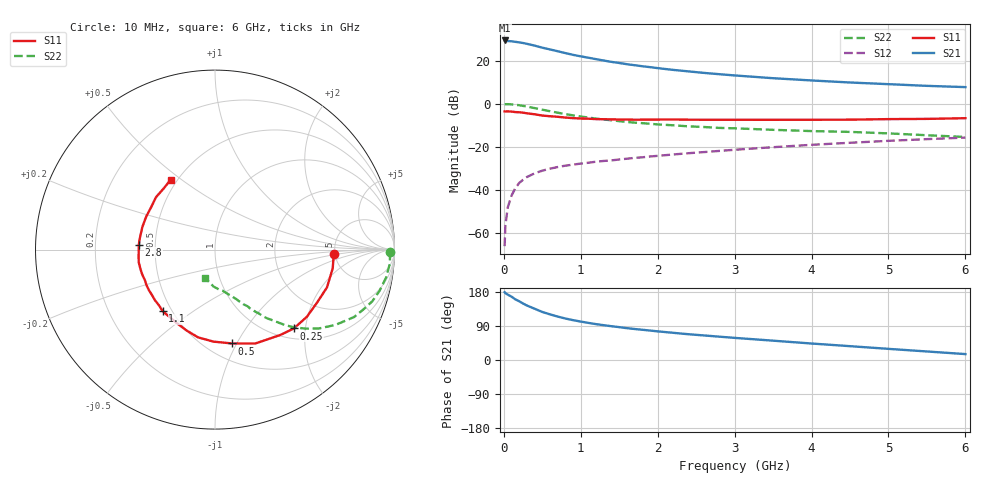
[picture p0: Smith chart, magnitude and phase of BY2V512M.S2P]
! SIEMENS Small Signal Semiconductors
! BFY420
! Si NPN RF SIEGET Grounded Emitter Transistor in MICRO-X
! VCE = 2.5 V  IC = 12 mA
! Common Emitter S-Parameters:  October  1996
# GHz  S  MA  R  50
!  f  S11  S21  S12  S22
! GHz  MAG  ANG  MAG  ANG  MAG  ANG  MAG  ANG
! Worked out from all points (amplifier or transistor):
!   36 points, 10 MHz to 6 GHz, reference 50 ohm
!   highest |S21| = 29.3 dB at 10 MHz (marker M1)
!   |S21| within 3 dB of that: start of sweep to 463.6 MHz
!   unconditionally stable (mu >= 1): 2.387 GHz to end of sweep
!   at 250 MHz: K = 0.22, MSG = 31.7 dB, |S12| = -35.2 dB
!   at 1.4 GHz: K = 0.80, MSG = 22.8 dB, |S12| = -26.2 dB
!   at 6 GHz: K = 1.09, MAG = 9.9 dB, |S12| = -15.7 dB
!   S11 on the Smith chart (normalised r, x): 10 MHz: 4.91, -0.43; 250 MHz: 1.21, -1.73; 500 MHz: 0.66, -0.96; 1.1 GHz: 0.45, -0.38; 2.8 GHz: 0.40, +0.03; 6 GHz: 0.46, +0.46
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0.01  0.664 -2.1  29.25 178.9  0.0005 91.6  0.9764 -0.7
0.02  0.6618 -3.6  29.09 176.5  0.0015 87.3  0.9755 -1.6
0.05  0.6642 -9.1  28.32 172.6  0.0039 86.6  0.9775 -4.6
0.1  0.6584 -18.7  27.97 167.1  0.0074 84.3  0.9654 -9.4
0.15  0.6407 -27.4  27.17 160.0  0.0111 77.5  0.9455 -14.0
0.2  0.6341 -36.2  26.43 155.0  0.0146 74.1  0.9225 -18.2
0.25  0.6213 -45.0  25.51 149.0  0.0173 69.3  0.8896 -22.2
0.3  0.5989 -52.6  24.44 143.8  0.02 68.3  0.8607 -25.9
0.4  0.5693 -66.8  22.2 135.3  0.0244 63.0  0.7917 -32.0
0.5  0.5317 -79.6  19.9 126.8  0.0281 59.5  0.7281 -37.1
0.6  0.5129 -90.9  18.11 120.4  0.0313 56.3  0.67 -41.1
0.8  0.4777 -109.4  14.9 109.5  0.0367 53.1  0.5745 -47.1
0.9  0.4633 -116.4  13.57 105.1  0.0388 52.8  0.5369 -49.1
1.1  0.45 -130.3  11.64 97.9  0.0429 51.8  0.4779 -53.0
1.3  0.4374 -140.0  10.01 91.8  0.0472 50.7  0.4303 -55.6
1.6  0.4301 -152.5  8.24 84.0  0.0532 50.7  0.3777 -59.4
2.2  0.4308 -170.6  6.085 71.8  0.0666 50.2  0.3165 -65.1
2.8  0.425 176.3  4.837 61.6  0.0806 48.2  0.2753 -70.2
3.5  0.4239 162.8  3.902 51.0  0.0983 44.8  0.2483 -75.8
4.5  0.4272 146.3  3.104 36.5  0.1245 38.2  0.2223 -84.8
5.5  0.4453 129.5  2.595 22.5  0.1511 30.0  0.1861 -98.9
6  0.462 122.3  2.426 15.6  0.1641 25.5  0.1696 -108.5
